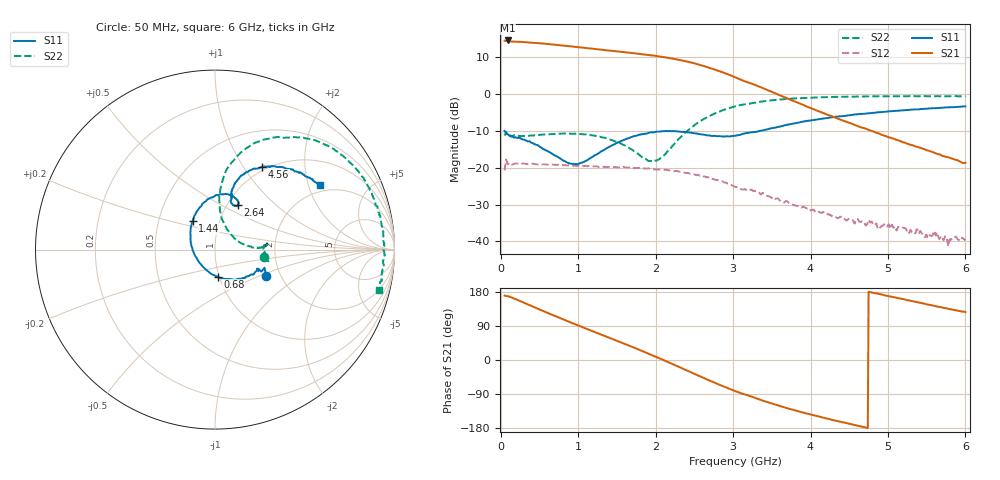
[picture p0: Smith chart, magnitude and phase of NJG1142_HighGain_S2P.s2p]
! Created Thu Jun  3 16:19:03 2010
# hz S ma R 50
! 2 Port Network Data from SP7.SP block
! freq  magS11  angS11  magS21  angS21  magS12  angS12  magS22  angS22
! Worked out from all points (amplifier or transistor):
!   596 points, 50 MHz to 6 GHz, reference 50 ohm
!   highest |S21| = 14.6 dB at 90 MHz (marker M1)
!   |S21| within 3 dB of that: start of sweep to 1.517 GHz
!   unconditionally stable (mu >= 1): start of sweep to end of sweep
!   at 1.04 GHz: K = 1.25, MAG = 13.1 dB, |S12| = -19.5 dB
!   at 3.03 GHz: K = 2.48, MAG = 8.1 dB, |S12| = -25.2 dB
!   at 6 GHz: K = 26.18, MAG = -6.7 dB, |S12| = -39.7 dB
!   lowest NFmin = 1.50 dB at 50 MHz
!   S11 on the Smith chart (normalised r, x): 50 MHz: 1.67, -0.55; 680 MHz: 0.98, -0.30; 1.44 GHz: 0.74, +0.25; 2.64 GHz: 1.12, +0.61; 4.56 GHz: 0.95, +1.22; 6 GHz: 1.73, +2.37
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5e7  0.318 -27.4  5.336 170.0  0.09205 0.8  0.2742 -8.5
9e7  0.2857 -25.4  5.383 168.4  0.1125 5.0  0.2653 -8.2
2.6e8  0.2509 -33.6  5.148 154.8  0.1132 -7.7  0.2695 0.8
4.8e8  0.2027 -55.9  4.955 135.1  0.1114 -17.3  0.2772 5.4
6.8e8  0.1511 -84.6  4.738 117.8  0.1106 -24.6  0.289 6.3
8.8e8  0.1159 -126.4  4.502 101.0  0.1086 -32.0  0.2923 6.1
1.05e9  0.118 -168.6  4.308 87.1  0.1062 -38.2  0.2874 4.8
1.21e9  0.147 158.3  4.135 74.2  0.1049 -44.6  0.2742 3.3
1.44e9  0.2033 127.9  3.89 55.3  0.1026 -53.3  0.2364 2.7
1.76e9  0.275 100.4  3.571 29.4  0.09914 -67.2  0.1587 11.1
1.88e9  0.292 92.2  3.453 19.2  0.09756 -72.9  0.1303 25.7
2.04e9  0.3107 82.4  3.269 5.3  0.09511 -81.2  0.13 58.1
2.2e9  0.3154 74.4  3.08 -9.0  0.09099 -90.3  0.1888 79.3
2.37e9  0.3069 67.6  2.829 -24.4  0.08621 -101.8  0.2903 85.3
2.64e9  0.2803 62.8  2.391 -49.2  0.07598 -118.5  0.4721 80.4
2.84e9  0.2681 65.2  2.031 -66.6  0.06637 -131.0  0.5927 72.7
3.03e9  0.2731 70.3  1.7 -82.1  0.05515 -143.8  0.685 64.3
3.48e9  0.342 73.9  1.104 -113.5  0.04032 -165.6  0.8251 47.7
4.02e9  0.4453 69.8  0.6402 -144.9  0.02689 166.6  0.9013 31.4
4.56e9  0.5296 60.4  0.3874 -171.0  0.01811 138.5  0.9283 18.5
5.01e9  0.5852 52.1  0.2601 168.6  0.01716 120.1  0.9375 8.2
6e9  0.6864 31.9  0.1172 126.3  0.01036 69.8  0.9395 -13.7
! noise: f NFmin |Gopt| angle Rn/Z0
5e+07  1.505  0.2084  13.48  0.2462
7.1e+08  1.588  0.1226  50.3  0.2059
1.37e+09  1.746  0.0888  -177.6  0.1636
2.03e+09  2.025  0.2758  -114.9  0.2125
2.69e+09  2.494  0.4483  -83.98  0.4755
3.35e+09  3.286  0.5559  -61.9  1.07
4.01e+09  4.567  0.6082  -46.36  2.171
4.67e+09  6.468  0.6455  -36.81  4.458
5.33e+09  8.587  0.7125  -28.63  10.35
6e+09  10.8  0.8098  -18.86  29.4
